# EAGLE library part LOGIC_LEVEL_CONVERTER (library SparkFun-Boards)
SparkFun Logic Level Converter -Bi-Directional This is the mechnical outline for the 3.3V - 5V bi directional logic level converter. SparkFun Products: SparkFun Logic Level Converter - Bi-Directional
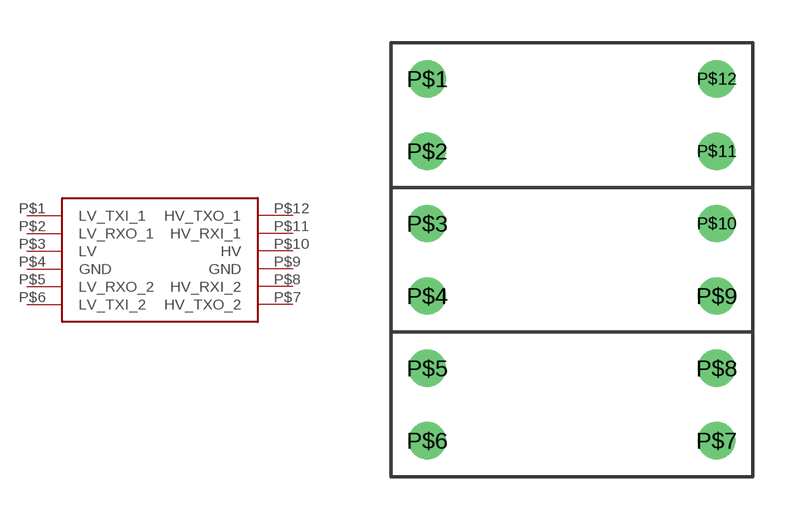
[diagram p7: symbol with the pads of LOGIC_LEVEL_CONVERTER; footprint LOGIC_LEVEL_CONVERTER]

Designator prefix B

## LOGIC_LEVEL_CONVERTER  [LOGIC_LEVEL_CONVERTER]
P$1  LV_TXI_1
P$2  LV_RXO_1
P$3  LV
P$4  GND
P$5  LV_RXO_2
P$6  LV_TXI_2
P$7  HV_TXO_2
P$8  HV_RXI_2
P$9  GND
P$10  HV
P$11  HV_RXI_1
P$12  HV_TXO_1

## Footprint LOGIC_LEVEL_CONVERTER (pad centres in mm)
drill 0.8: P$1 1.27,13.97; P$2 1.27,11.43; P$3 1.27,8.89; P$4 1.27,6.35; P$5 1.27,3.81; P$6 1.27,1.27; P$7 11.43,1.27; P$8 11.43,3.81; P$9 11.43,6.35; P$10 11.43,8.89; P$11 11.43,11.43; P$12 11.43,13.97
